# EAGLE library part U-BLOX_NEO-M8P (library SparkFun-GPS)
U-blox NEO-M8P The NEO-M8P module combines the high performance u-blox M8 positioning engine with u-blox’s Real Time Kinematic (RTK) technology. The NEO-M8P provides cm-level GNSS performance designed to meet the needs of unmanned vehicles and other machine control applications requiring high precision guidance.
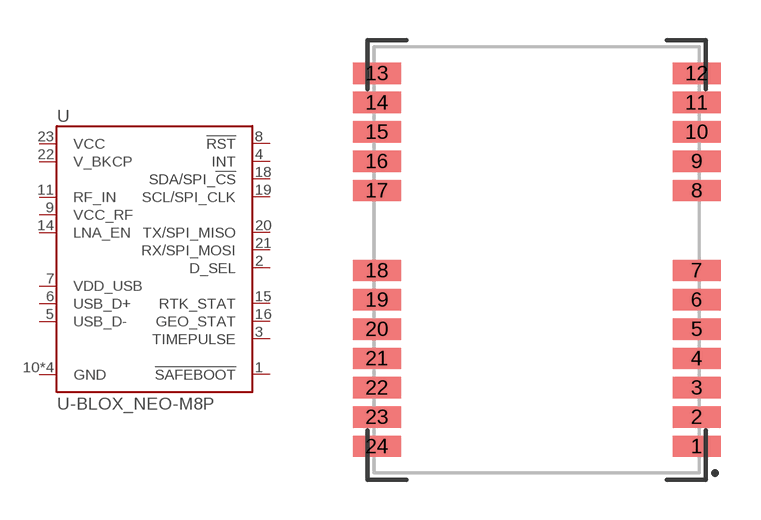
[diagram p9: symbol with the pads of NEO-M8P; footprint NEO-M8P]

Designator prefix U

## U-BLOX_NEO-M8PM8P (PROD_ID: IC-14069)  [NEO-M8P]
1  !SAFEBOOT!
2  D_SEL
3  TIMEPULSE
4  INT
5  USB_D-
6  USB_D+
7  VDD_USB
8  !RST
9  VCC_RF
10  GND
11  RF_IN
12  GND
13  GND
14  LNA_EN
15  RTK_STAT
16  GEO_STAT
18  SDA/SPI_!CS!
19  SCL/SPI_CLK
20  TX/SPI_MISO
21  RX/SPI_MOSI
22  V_BKCP
23  VCC
24  GND

## Footprint NEO-M8P (pad centres in mm)
smd 1.8 x 0.8: 1 6,-7; 2 6,-5.9; 3 6,-4.8; 4 6,-3.7; 5 6,-2.6; 6 6,-1.5; 7 6,-0.4; 8 6,2.6; 9 6,3.7; 10 6,4.8; 11 6,5.9; 12 6,7; 13 -6,7; 14 -6,5.9; 15 -6,4.8; 16 -6,3.7; 17 -6,2.6; 18 -6,-0.4; 19 -6,-1.5; 20 -6,-2.6; 21 -6,-3.7; 22 -6,-4.8; 23 -6,-5.9; 24 -6,-7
